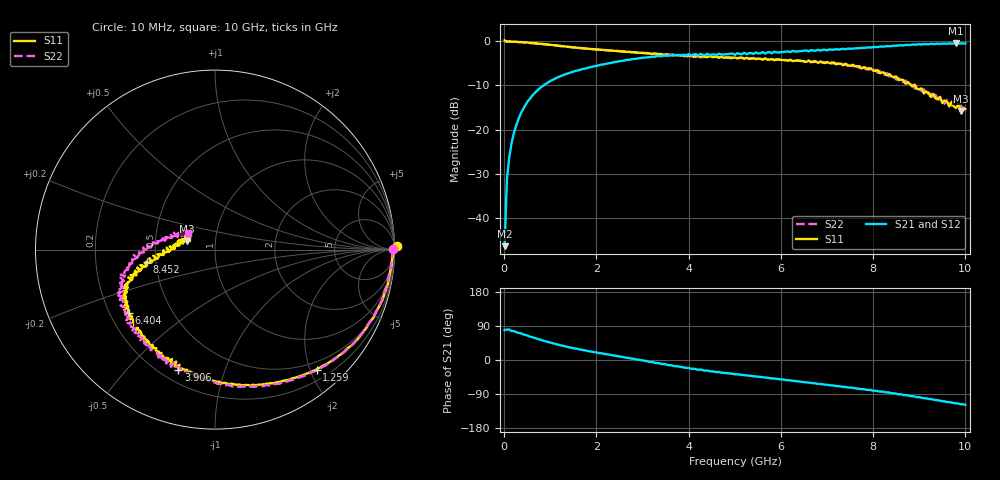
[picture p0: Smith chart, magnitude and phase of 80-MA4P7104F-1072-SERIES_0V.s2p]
!Agilent Technologies,E8364C,MY48140145,A.09.42.15
!Agilent E8364C: A.09.42.15
!Date: Wednesday, December 02, 2020 07:32:53
!Correction: S11(Full 2 Port(1,2))
!S21(Full 2 Port(1,2))
!S12(Full 2 Port(1,2))
!S22(Full 2 Port(1,2))
!S2P File: Measurements: S11, S21, S12, S22:
# Hz S  dB  R 50
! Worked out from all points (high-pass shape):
!   201 points, 10 MHz to 10 GHz, reference 50 ohm
!   highest |S21| = -0.53 dB at 9.8 GHz (marker M1); lowest = -46.3 dB at 10 MHz (marker M2)
!   |S21| within 3 dB of the highest: 3.266 GHz to end of sweep
!   lowest |S11| = -15.8 dB at 9.9 GHz (marker M3), VSWR 1.39, Z = 36.4 + j3.49 ohm
!   |S11| at or under -10 dB: 8.825 GHz to 8.882 GHz (56.97 MHz wide, 0.643 % of centre); 8.91 GHz to end of sweep
!   |S22| runs from -15.6 to -0.1 dB; largest |S21 - S12| = 0.024
!   S11 on the Smith chart (normalised r, x): 10 MHz: -45, +67; 1.259 GHz: 0.37, -2.10; 3.906 GHz: 0.27, -0.71; 6.404 GHz: 0.28, -0.30; 8.452 GHz: 0.44, -0.07; 10 GHz: 0.72, +0.10
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1e7  0.12 1.2  -46.29 79.2  -44.18 28.0  -0.06 0.3
5.995e7  -0.11 -2.9  -31.19 80.3  -31.40 79.4  -0.13 -3.0
1.099e8  -0.11 -5.2  -26.29 80.4  -26.26 79.8  -0.14 -5.3
1.5985e8  -0.15 -7.6  -23.10 76.5  -23.11 76.6  -0.18 -7.7
2.5975e8  -0.18 -12.4  -19.09 73.8  -19.08 73.9  -0.22 -12.6
6.094e8  -0.45 -27.1  -12.32 60.2  -12.31 60.4  -0.48 -27.9
1.25875e9  -1.16 -49.7  -7.78 37.7  -7.77 37.7  -1.19 -51.5
1.7083e9  -1.65 -61.8  -6.30 26.3  -6.29 26.4  -1.63 -64.2
3.35665e9  -2.94 -97.1  -3.40 -8.2  -3.37 -9.1  -2.99 -100.0
3.9061e9  -3.11 -106.9  -3.19 -20.0  -3.12 -19.7  -3.47 -110.2
5.005e9  -3.72 -122.6  -3.15 -37.8  -3.09 -37.0  -3.68 -129.5
6.4036e9  -4.49 -143.7  -2.29 -56.8  -2.28 -56.8  -4.43 -149.8
6.7033e9  -4.74 -148.8  -2.17 -61.1  -2.16 -60.9  -4.48 -154.6
7.9021e9  -6.45 -162.9  -1.45 -79.0  -1.50 -78.9  -6.06 -171.1
8.35165e9  -7.43 -168.2  -1.18 -86.0  -1.14 -86.9  -8.03 -177.6
8.45155e9  -8.24 -170.1  -1.06 -87.8  -1.11 -88.4  -7.97 -179.3
9.2008e9  -11.75 -177.3  -0.73 -102.8  -0.68 -102.1  -11.64 159.3
9.75025e9  -14.79 169.4  -0.58 -113.7  -0.56 -113.0  -13.70 150.1
9.8002e9  -15.12 160.4  -0.53 -114.1  -0.57 -114.4  -14.92 154.7
9.85015e9  -14.18 163.2  -0.60 -115.1  -0.54 -115.2  -14.65 145.6
9.9001e9  -15.78 163.3  -0.55 -116.6  -0.56 -116.2  -14.36 151.7
1e10  -15.38 157.3  -0.55 -118.2  -0.55 -118.2  -15.06 148.2
